(* Logix 5000 AddOnInstructionDefinition export AMCI_SMD34E2_Preset_Motor_to_Encoder; software revision 20.03 *)

ADD_ON_INSTRUCTION AMCI_SMD34E2_Preset_Motor_to_Encoder   (* revision 1.0, vendor AMCI *)
VAR_IN_OUT
   AMCI_SMD34E2_output_data : _000A:SMD34E2_788832CB:O:0; {required}
END_VAR
VAR
   Upper_Result_X_1000 : DINT;
   command_data_block : INT[10];
        [0]   // Command Bits MSW
        [1]   // Command Bits LSW
        [2]   // Upper Target Position
        [3]   // Lower Target Position
        [4]   // Upper Programmed Speed
        [5]   // Lower Programmed Speed
END_VAR

ROUTINE Logic   (* ladder *)
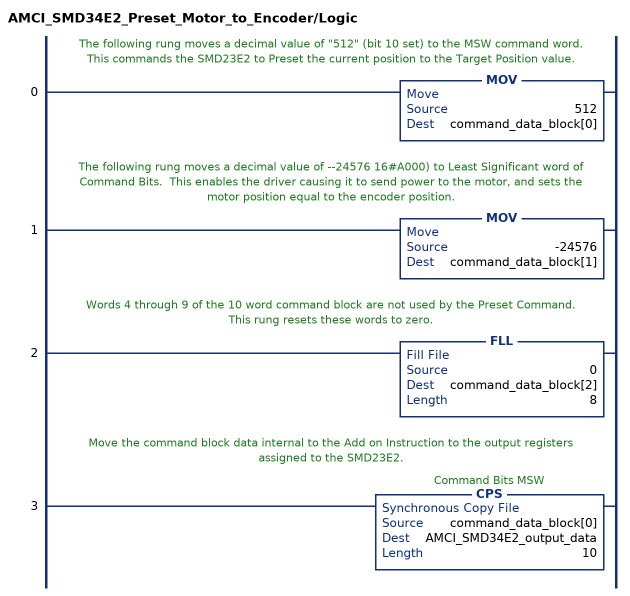
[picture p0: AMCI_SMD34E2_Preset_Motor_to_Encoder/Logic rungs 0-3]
   // The following rung moves a decimal value of "512" (bit 10 set) to the MSW command word.  This commands the SMD23E2 to Preset the current position to the Target Position value.
   0: MOV(512,command_data_block[0]);
   // The following rung moves a decimal value of --24576 16#A000) to Least Significant word of Command Bits.  This enables the driver causing it to send power to the motor, and sets the motor position equal to the encoder position.
   1: MOV(-24576,command_data_block[1]);
   // Words 4 through 9 of the 10 word command block are not used by the Preset Command.  This rung resets these words to zero.
   2: FLL(0,command_data_block[2],8);
   // Move the command block data internal to the Add on Instruction to the output registers assigned to the SMD23E2.
   3: CPS(command_data_block[0],AMCI_SMD34E2_output_data,10);
END_ROUTINE
END_ADD_ON_INSTRUCTION
